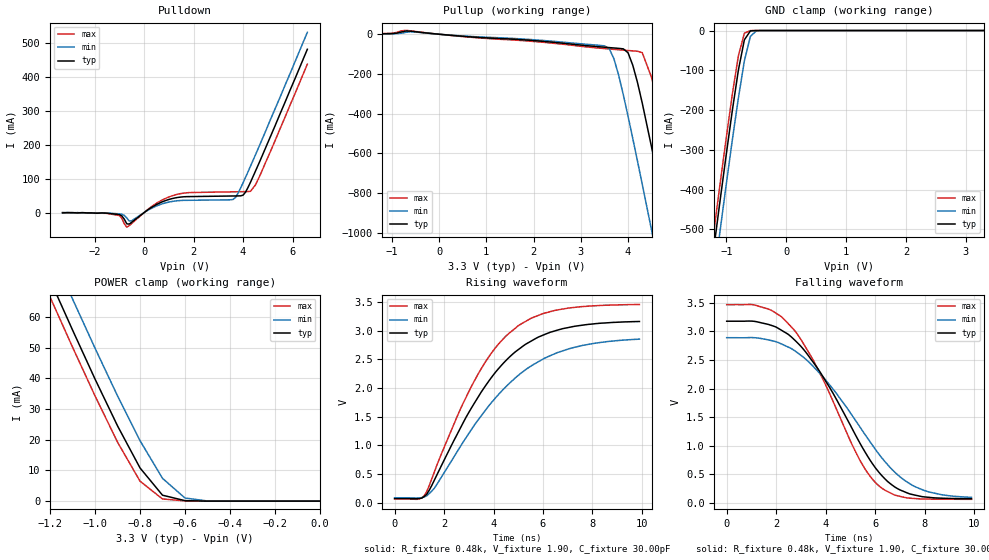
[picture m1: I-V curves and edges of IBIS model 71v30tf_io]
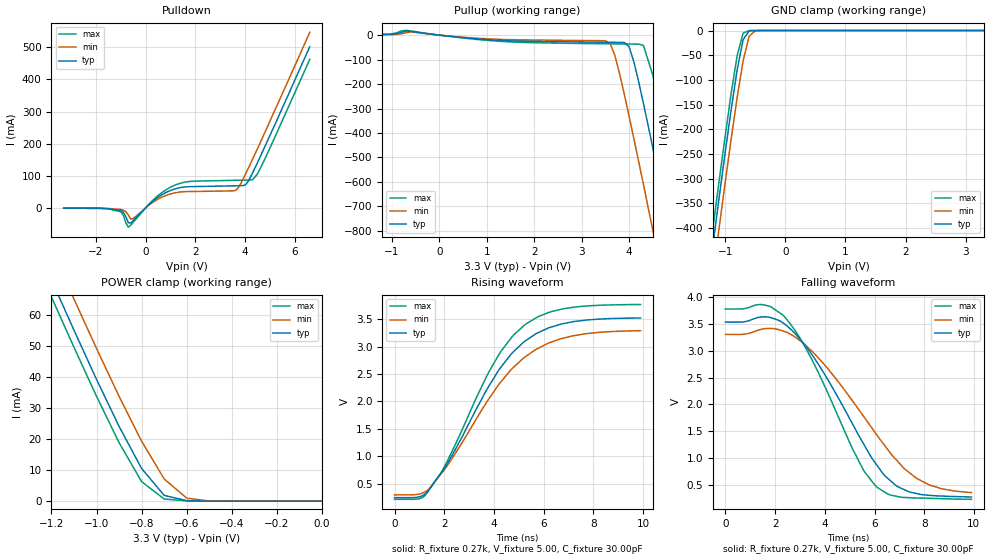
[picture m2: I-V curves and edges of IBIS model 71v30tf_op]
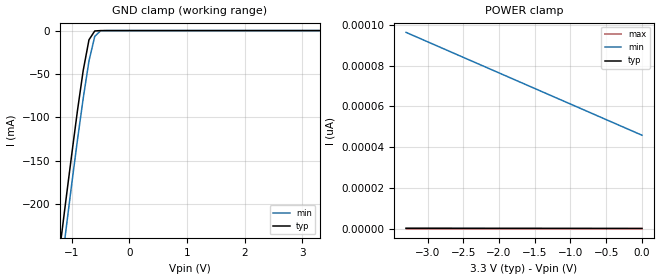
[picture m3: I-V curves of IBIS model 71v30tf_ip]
| IBIS file 71v30tf.ibs created by s2ibis2 version 1.1
| North Carolina State University Electronics Research Laboratory  1995
[IBIS ver]   2.1
[File name]   71v30tf.ibs
[File Rev]   1.0
[Date]   12/13/99
[Source]   Integrated Device Technology, Inc.
[Notes]   1.Temperatures: typ=25C, min=70C, max=0C 2.Cemos7_5v process.
   3.RRmp rates based on 50 ohm load.
[Disclaimer]   This information is for modeling purpose only, and is not
   guaranteed.
[Copyright]   Copyright 1999, Integrated Device Technology, Inc. all rights
   reserved
|   Component 71v30tf
[Component]   71v30tf
[Manufacturer]   Integrated Device Technology
[Package]
| variable   typ   min   max
R_pkg   50.00m   50.00m   50.00m
L_pkg   4.50nH   4.23nH   4.78nH
C_pkg   0.14pF   0.12pF   0.16pF
[Pin]  signal_name   model_name   R_pin   L_pin   C_pin
1   OEL   71v30tf_ip
2   A0L   71v30tf_ip
3   A1L   71v30tf_ip
4   A2L   71v30tf_ip
5   A3L   71v30tf_ip
6   A4L   71v30tf_ip
7   A5L   71v30tf_ip
8   A6L   71v30tf_ip
9   NC   NC
10   A7L   71v30tf_ip
11   A8L   71v30tf_ip
12   A9L   71v30tf_ip
13   NC   NC
14   IO0L   71v30tf_io
15   IO1L   71v30tf_io
16   IO2L   71v30tf_io
17   IO3L   71v30tf_io
18   NC   NC
19   IO4L   71v30tf_io
20   IO5L   71v30tf_io
21   IO6L   71v30tf_io
22   IO7L   71v30tf_io
23   NC   NC
24   GND   GND
25   GND   GND
26   IO0R   71v30tf_io
27   IO1R   71v30tf_io
28   IO2R   71v30tf_io
29   IO3R   71v30tf_io
30   NC   NC
31   IO4R   71v30tf_io
32   IO5R   71v30tf_io
33   IO6R   71v30tf_io
34   IO7R   71v30tf_io
35   NC   NC
36   NC   NC
37   A9R   71v30tf_ip
38   A8R   71v30tf_ip
39   A7R   71v30tf_ip
40   NC   NC
41   A6R   71v30tf_ip
42   A5R   71v30tf_ip
43   A4R   71v30tf_ip
44   A3R   71v30tf_ip
45   A2R   71v30tf_ip
46   A1R   71v30tf_ip
47   A0R   71v30tf_ip
48   OER   71v30tf_ip
49   NC   NC
50   NC   NC
51   NC   NC
52   INTR   71v30tf_op
53   BUSYR   71v30tf_op
54   RWR   71v30tf_ip
55   CER   71v30tf_ip
56   VCC   POWER
57   VCC   POWER
58   CEL   71v30tf_ip
59   RWL   71v30tf_ip
60   BUSYL   71v30tf_op
61   INTL   71v30tf_op
62   NC   NC
63   NC   NC
64   NC   NC
| Models and submodels in the file (3): 71v30tf_io (I/O), 71v30tf_op (3-state), 71v30tf_ip (Input)
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| in   in   dummy
| oeh  oeh   dummy
|   Model 71v30tf_io
[Model]   71v30tf_io
Model_type   I/O
Polarity   Non-Inverting
Enable   Active-High
Vinl =  0.800V
Vinh =  2.000V
Vmeas =  1.500V
C_comp   3.00pF   NA   NA
[Temperature Range]   25.00   70.00   0.000
[Voltage Range]   3.30V   3.00V   3.60V
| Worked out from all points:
|   slope of the pulldown table from 0 to 0.495 V, typ, clamps not added: 21.1 ohm
|   slope of the pullup table from 0 to 0.495 V, typ, clamps not added: 48.5 ohm
|   GND clamp passes 1 mA (typ) near -0.60 V on its own axis
|   POWER clamp passes 1 mA (typ) near -0.65 V on its own axis
|   rising waveform, R_fixture 0.48k, V_fixture 1.90, C_fixture 30.00pF: 20-80 % time 2.71ns typ, 3.06ns min, 2.43ns max; typ from 0.069 V to 3.16 V
|   falling waveform, R_fixture 0.48k, V_fixture 1.90, C_fixture 30.00pF: 20-80 % time 2.55ns typ, 2.91ns min, 2.29ns max; typ from 3.18 V to 0.077 V
[Pulldown]
| voltage   I(typ)   I(min)   I(max)
-3.3V     -1mA       0A         0A
-1V       -5.9mA     -3.7mA     -8.9mA
-700mV    -33.32mA   -16.01mA   -43.03mA
-500mV    -28.4mA    -23.83mA   -32.06mA
400mV     19.69mA    16.29mA    22.7mA
1.1V      40.7mA     32.45mA    48.65mA
1.8V      47.13mA    36.23mA    58.84mA
3.6V      48.97mA    38.76mA    61.24mA
4V        51.3mA     87.79mA    61.7mA
4.3V      89.34mA    137mA      62.75mA
4.5V      122mA      170mA      81.44mA
6.6V      482mA      532mA      438mA
[Pullup]
| voltage   I(typ)   I(min)   I(max)
-3.3V     200uA      200uA      300uA
-700mV    16.39mA    9.535mA    19.42mA
3.5V      -65.34mA   -58.45mA   -72.24mA
3.7V      -69.19mA   -123mA     -76.26mA
4V        -93.34mA   -413mA     -81.98mA
4.3V      -346mA     -755mA     -92.73mA
4.5V      -571mA     -989mA     -219mA
4.7V      -803mA     -1.226A    -423mA
4.9V      -1.039A    -1.464A    -652mA
5.1V      -1.277A    -1.703A    -886mA
5.3V      -1.516A    -1.943A    -1.123A
6.6V      -3.085A    -3.513A    -2.689A
[GND_clamp]
| voltage   I(typ)   I(min)   I(max)
-3.3V     -3.052A    -3.124A    -3.013A
-1.3V     -652mA     -728mA     -610mA
-1.2V     -536mA     -612mA     -494mA
-1.1V     -421mA     -497mA     -379mA
-1V       -309mA     -384mA     -267mA
-900mV    -200mA     -274mA     -159mA
-800mV    -99.72mA   -170mA     -63.69mA
-700mV    -23.46mA   -76.46mA   -6.732mA
-600mV    -1.049mA   -15.04mA   -119uA
-500mV    -20.56uA   -807uA     -1.708uA
3.3V      77.38fA    39.44nA    -39.89fA
[POWER_clamp]
| voltage   I(typ)   I(min)   I(max)
-3.3V     430mA      440mA      425mA
-1.2V     71.89mA    82.02mA    66.32mA
-1.1V     55.61mA    65.72mA    50.03mA
-1V       39.67mA    49.72mA    34.19mA
-900mV    24.47mA    34.23mA    19.17mA
-800mV    10.8mA     19.68mA    6.49mA
-700mV    1.935mA    7.435mA    707uA
-600mV    161uA      1.022mA    71.85uA
-500mV    961nA      56.33uA    81.5nA
0V        57.04fA    96.11pA    828fA
[Ramp]
| variable   typ   min   max
dV/dt_r   0.87/0.68n   0.73/0.96n   1.03/0.55n
dV/dt_f   1.22/3.01n   0.98/3.34n   1.44/2.68n
R_load = 50.00
[Rising Waveform]
R_fixture = 0.48k
V_fixture = 1.90
C_fixture = 30.00pF
R_dut = 50.00m
L_dut = 4.50nH
C_dut = 0.14pF
| time   V(typ)   V(min)   V(max)
0s        69.44mV    82.31mV    61.31mV
1.2ns     106mV      100mV      121mV
1.6ns     385mV      246mV      524mV
2.6ns     1.251V     938mV      1.574V
3.3ns     1.789V     1.398V     2.185V
4.1ns     2.288V     1.839V     2.717V
5ns       2.672V     2.222V     3.09V
5.8ns     2.889V     2.458V     3.268V
7.1ns     3.065V     2.693V     3.402V
9.9ns     3.164V     2.856V     3.461V
[Falling Waveform]
R_fixture = 0.48k
V_fixture = 1.90
C_fixture = 30.00pF
R_dut = 50.00m
L_dut = 4.50nH
C_dut = 0.14pF
| time   V(typ)   V(min)   V(max)
0s        3.177V     2.889V     3.466V
1.7ns     3.119V     2.849V     3.387V
2.7ns     2.868V     2.676V     3.039V
3.8ns     2.273V     2.251V     2.24V
5.4ns     1.038V     1.323V     739mV
6.2ns     516mV      830mV      285mV
6.8ns     281mV      539mV      139mV
7.6ns     141mV      291mV      80.18mV
8.7ns     85.93mV    146mV      68.57mV
9.9ns     76.64mV    101mV      66.09mV
|   Model 71v30tf_op
[Model]   71v30tf_op
Model_type   3-state
Polarity   Non-Inverting
Enable   Active-High
Vinl =  0.800V
Vinh =  2.000V
Vmeas =  1.500V
C_comp   3.00pF   NA   NA
[Temperature Range]   25.00   70.00   0.000
[Voltage Range]   3.30V   3.00V   3.60V
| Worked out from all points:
|   slope of the pulldown table from 0 to 0.495 V, typ, clamps not added: 15 ohm
|   slope of the pullup table from 0 to 0.495 V, typ, clamps not added: 48.5 ohm
|   GND clamp passes 1 mA (typ) near -0.60 V on its own axis
|   POWER clamp passes 1 mA (typ) near -0.65 V on its own axis
|   rising waveform, R_fixture 0.27k, V_fixture 5.00, C_fixture 30.00pF: 20-80 % time 2.53ns typ, 2.73ns min, 2.39ns max; typ from 0.242 V to 3.53 V
|   falling waveform, R_fixture 0.27k, V_fixture 5.00, C_fixture 30.00pF: 20-80 % time 2.46ns typ, 2.89ns min, 2.16ns max; typ from 3.53 V to 0.277 V
[Pulldown]
| voltage   I(typ)   I(min)   I(max)
-3.3V     -1mA       -1mA       -1mA
-1V       -8.4mA     -5.2mA     -12.4mA
-700mV    -46.75mA   -22.48mA   -60.3mA
-500mV    -39.76mA   -33.38mA   -44.88mA
400mV     27.56mA    22.8mA     31.77mA
1.1V      56.99mA    45.43mA    68.11mA
1.8V      65.99mA    50.73mA    82.38mA
3.6V      68.57mA    53.8mA     85.75mA
4V        70.97mA    103mA      86.39mA
4.3V      109mA      152mA      87.55mA
4.5V      141mA      185mA      106mA
6.6V      502mA      547mA      463mA
[Pullup]
| voltage   I(typ)   I(min)   I(max)
-3.3V     300uA      200uA      300uA
-700mV    16.47mA    9.742mA    19.45mA
3.5V      -29.1mA    -23.46mA   -35.46mA
3.7V      -29.43mA   -83.98mA   -35.86mA
4V        -48.3mA    -333mA     -36.38mA
4.3V      -279mA     -610mA     -42.04mA
4.5V      -462mA     -800mA     -165mA
4.7V      -651mA     -991mA     -343mA
4.9V      -842mA     -1.183A    -529mA
5.1V      -1.033A    -1.376A    -719mA
5.3V      -1.226A    -1.57A     -911mA
6.6V      -2.492A    -2.836A    -2.174A
[GND_clamp]
| voltage   I(typ)   I(min)   I(max)
-3.3V     -2.46A     -2.518A    -2.429A
-1.3V     -525mA     -587mA     -492mA
-1.2V     -432mA     -493mA     -398mA
-1.1V     -339mA     -400mA     -305mA
-1V       -248mA     -309mA     -215mA
-900mV    -161mA     -220mA     -128mA
-800mV    -79.81mA   -136mA     -50.96mA
-700mV    -18.44mA   -60.81mA   -5.207mA
-600mV    -744uA     -11.53mA   -92.46uA
-500mV    -15.57uA   -544uA     -1.326uA
3.3V      -214fA     36.28nA    -370fA
[POWER_clamp]
| voltage   I(typ)   I(min)   I(max)
-3.3V     430mA      439mA      425mA
-1.2V     71.53mA    81.6mA     65.99mA
-1.1V     55.25mA    65.31mA    49.71mA
-1V       39.33mA    49.32mA    33.89mA
-900mV    24.15mA    33.86mA    18.89mA
-800mV    10.54mA    19.35mA    6.295mA
-700mV    1.846mA    7.158mA    683uA
-600mV    158uA      968uA      71.42uA
-500mV    884nA      53.68uA    75nA
0V        675fA      76.32pA    366fA
[Ramp]
| variable   typ   min   max
dV/dt_r   0.77/1.60n   0.60/1.70n   0.94/1.53n
dV/dt_f   1.42/2.72n   1.19/3.14n   1.64/2.38n
R_load = 50.00
[Rising Waveform]
R_fixture = 0.27k
V_fixture = 5.00
C_fixture = 30.00pF
R_dut = 50.00m
L_dut = 4.50nH
C_dut = 0.14pF
| time   V(typ)   V(min)   V(max)
0s        242mV      293mV      211mV
1ns       257mV      306mV      222mV
1.3ns     340mV      366mV      322mV
2ns       769mV      751mV      801mV
3.7ns     2.209V     1.984V     2.455V
4.2ns     2.579V     2.315V     2.857V
5.3ns     3.119V     2.83V      3.42V
6.2ns     3.346V     3.069V     3.626V
7.2ns     3.46V      3.203V     3.723V
9.9ns     3.527V     3.295V     3.773V
[Falling Waveform]
R_fixture = 0.27k
V_fixture = 5.00
C_fixture = 30.00pF
R_dut = 50.00m
L_dut = 4.50nH
C_dut = 0.14pF
| time   V(typ)   V(min)   V(max)
0s        3.531V     3.302V     3.775V
1.5ns     3.626V     3.403V     3.855V
2.4ns     3.488V     3.353V     3.619V
3.1ns     3.16V      3.149V     3.154V
3.9ns     2.63V      2.783V     2.435V
5.5ns     1.314V     1.817V     827mV
6.1ns     867mV      1.427V     458mV
6.9ns     478mV      956mV      289mV
7.7ns     341mV      621mV      259mV
9.9ns     277mV      360mV      234mV
|   Model 71v30tf_ip
[Model]   71v30tf_ip
Model_type   Input
Vinl =  0.800V
Vinh =  2.000V
Vmeas =  1.500V
C_comp   3.00pF   NA   NA
[Temperature Range]   25.00   70.00   0.000
[Voltage Range]   3.30V   3.00V   3.60V
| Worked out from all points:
|   GND clamp passes 1 mA (typ) near -0.61 V on its own axis
[GND_clamp]
| voltage   I(typ)   I(min)   I(max)
-3.3V     -1.413A    -1.446A    NA
-1.2V     -248mA     -283mA     NA
-1.1V     -195mA     -230mA     NA
-1V       -143mA     -177mA     NA
-900mV    -92.23mA   -126mA     NA
-800mV    -45.82mA   -77.94mA   NA
-700mV    -10.61mA   -34.92mA   NA
-600mV    -443uA     -6.653mA   NA
-500mV    -9.504uA   -325uA     NA
-400mV    -194nA     -11.45uA   NA
3.3V      111fA      50.46pA    NA
[POWER_clamp]
| voltage   I(typ)   I(min)   I(max)
-3.3V     221fA      96.34pA    3.303fA
-2.3V     188fA      81.04pA    2.465fA
-1.1V     148fA      62.7pA     2.017fA
0V        111fA      45.87pA    1.597fA
